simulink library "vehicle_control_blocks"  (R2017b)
settings: Solver=ode1  StartTime=0.0  StopTime=Inf  FixedStep=0.001  RelTol=1e-3  EnableMultiTasking=on
PostLoadFcn:
  | , if any(exist('dsrtsu_mdlpostloadfcn', 'file') == [2, 3, 6]), try dsrtsu_mdlpostloadfcn('Execute', bdroot); catch fprintf('Error in PostLoadFcn (dsrtsu_mdlpostloadfcn) for model "%s":\n %s\n', bdroot, lasterr); end, end,
undefined symbols (not defined in the file or in its folder): ACCEL_KI, ACCEL_KP, ACCEL_MAX, ACCEL_TAU, ACCEL_TS, BRAKE_DEADBAND, DECEL_MAX, FUEL_CAPACITY, GAS_DENSITY, MAX_LATERAL_ACCEL, MAX_STEERING_WHEEL_ANGLE, MIN_SPEED, SPEED_KI, SPEED_KP, SPEED_TS, STEER_KP, STEERING_RATIO, VEHICLE_MASS, WHEEL_RADIUS, WHEELBASE
libraries: simulink x5

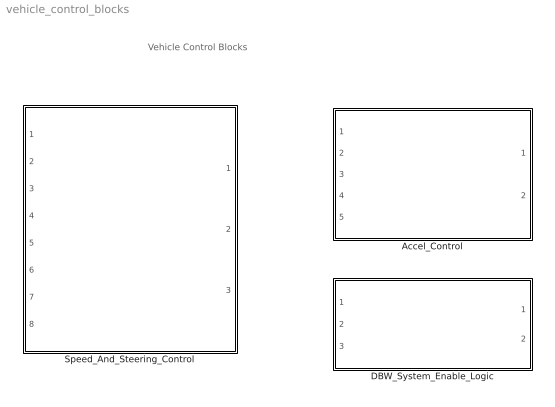
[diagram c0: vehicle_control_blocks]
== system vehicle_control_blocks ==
  note: Vehicle Control Blocks
  Accel_Control : Subsystem  InitFcn=accel_controller_config_init
  DBW_System_Enable_Logic : Subsystem
  Speed_And_Steering_Control : Subsystem  InitFcn=speed_controller_config_init

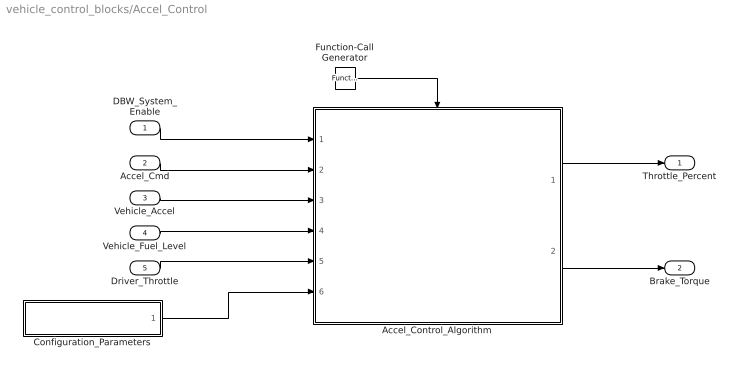
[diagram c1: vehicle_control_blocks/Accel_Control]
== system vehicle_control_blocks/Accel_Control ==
  DBW_System_Enable : Inport
  Accel_Cmd : Inport  Port=2
  Vehicle_Accel : Inport  Port=3
  Vehicle_Fuel_Level : Inport  Port=4
  Driver_Throttle : Inport  Port=5
  Accel_Control_Algorithm : Subsystem
  Configuration_Parameters : Subsystem
  Function-Call Generator : simulink/Ports & Subsystems/Function-Call Generator  sample_time=ACCEL_TS  numberOfIterations=1
  Throttle_Percent : Outport
  Brake_Torque : Outport  Port=2
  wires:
  Configuration_Parameters/1(Calibration_Parameters_Bus) -> Accel_Control_Algorithm/6(Calibration_Parameters_Bus)
  Vehicle_Fuel_Level/1 -> Accel_Control_Algorithm/4(Vehicle_Fuel_Level)
  Accel_Control_Algorithm/1(Throttle_Percent) -> Throttle_Percent/1
  Accel_Control_Algorithm/2(Brake_Torque) -> Brake_Torque/1
  Accel_Cmd/1 -> Accel_Control_Algorithm/2(Accel_Cmd)
  Vehicle_Accel/1 -> Accel_Control_Algorithm/3(Vehicle_Accel)
  Function-Call Generator/1 -> Accel_Control_Algorithm/Trigger
  DBW_System_Enable/1 -> Accel_Control_Algorithm/1(DBW_System_Enable)
  Driver_Throttle/1 -> Accel_Control_Algorithm/5(Driver_Throttle)

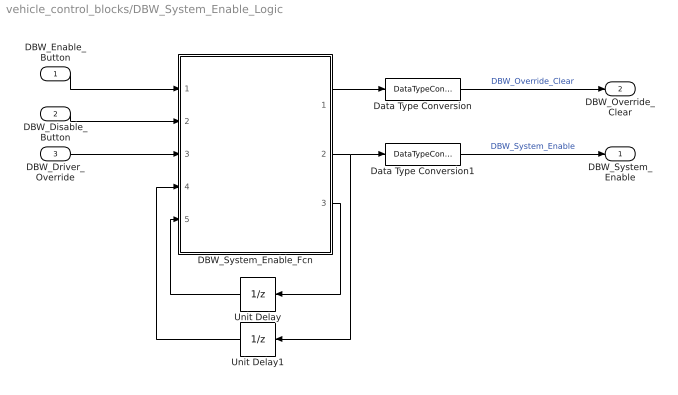
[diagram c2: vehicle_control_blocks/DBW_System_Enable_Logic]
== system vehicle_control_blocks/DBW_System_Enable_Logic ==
  DBW_Enable_Button : Inport
  DBW_Disable_Button : Inport  Port=2
  DBW_Driver_Override : Inport  Port=3
  DBW_System_Enable_Fcn : MATLAB Function  TreatAsAtomicUnit=on
  Data Type Conversion : DataTypeConversion  OutDataTypeStr=boolean
  Data Type Conversion1 : DataTypeConversion  OutDataTypeStr=boolean
  Unit Delay : UnitDelay  SampleTime=-1
  Unit Delay1 : UnitDelay  SampleTime=-1
  DBW_System_Enable : Outport
  DBW_Override_Clear : Outport  Port=2
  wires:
  DBW_Enable_Button/1 -> DBW_System_Enable_Fcn/1(enable_button)
  DBW_Disable_Button/1 -> DBW_System_Enable_Fcn/2(disable_button)
  DBW_Driver_Override/1 -> DBW_System_Enable_Fcn/3(driver_override)
  DBW_System_Enable_Fcn/3(state) -> Unit Delay/1
  DBW_System_Enable_Fcn/2(enable) -> Unit Delay1/1, Data Type Conversion1/1
  Unit Delay/1 -> DBW_System_Enable_Fcn/5(state_prev)
  Unit Delay1/1 -> DBW_System_Enable_Fcn/4(enable_prev)
  DBW_System_Enable_Fcn/1(clear_override) -> Data Type Conversion/1
  Data Type Conversion/1 -> DBW_Override_Clear/1  "DBW_Override_Clear"
  Data Type Conversion1/1 -> DBW_System_Enable/1  "DBW_System_Enable"

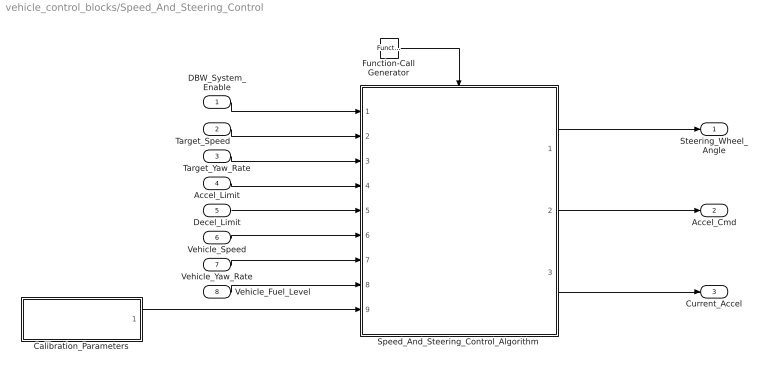
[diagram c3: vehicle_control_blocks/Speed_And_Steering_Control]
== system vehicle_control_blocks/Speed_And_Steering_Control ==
  DBW_System_Enable : Inport
  Target_Speed : Inport  Port=2
  Target_Yaw_Rate : Inport  Port=3
  Accel_Limit : Inport  Port=4
  Decel_Limit : Inport  Port=5
  Vehicle_Speed : Inport  Port=6
  Vehicle_Yaw_Rate : Inport  Port=7
  Vehicle_Fuel_Level : Inport  Port=8
  Calibration_Parameters : Subsystem
  Function-Call Generator : simulink/Ports & Subsystems/Function-Call Generator  sample_time=SPEED_TS  numberOfIterations=1
  Speed_And_Steering_Control_Algorithm : Subsystem
  Steering_Wheel_Angle : Outport
  Accel_Cmd : Outport  Port=2
  Current_Accel : Outport  Port=3
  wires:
  Calibration_Parameters/1(Calibration_Parameters_Bus) -> Speed_And_Steering_Control_Algorithm/9(Calibration_Parameters_Bus)
  Speed_And_Steering_Control_Algorithm/2(Accel_Cmd) -> Accel_Cmd/1
  Target_Speed/1 -> Speed_And_Steering_Control_Algorithm/2(Target_Speed)
  Target_Yaw_Rate/1 -> Speed_And_Steering_Control_Algorithm/3(Target_Yaw_Rate)
  Vehicle_Speed/1 -> Speed_And_Steering_Control_Algorithm/6(Vehicle_Speed)
  Speed_And_Steering_Control_Algorithm/1(Steering_Wheel_Angle) -> Steering_Wheel_Angle/1
  Vehicle_Yaw_Rate/1 -> Speed_And_Steering_Control_Algorithm/7(Vehicle_Yaw_Rate)
  Function-Call Generator/1 -> Speed_And_Steering_Control_Algorithm/Trigger
  Speed_And_Steering_Control_Algorithm/3(Current_Accel) -> Current_Accel/1
  Accel_Limit/1 -> Speed_And_Steering_Control_Algorithm/4(Accel_Limit)
  Decel_Limit/1 -> Speed_And_Steering_Control_Algorithm/5(Decel_Limit)
  DBW_System_Enable/1 -> Speed_And_Steering_Control_Algorithm/1(DBW_System_Enable)
  Vehicle_Fuel_Level/1 -> Speed_And_Steering_Control_Algorithm/8(Vehicle_Fuel_Level)

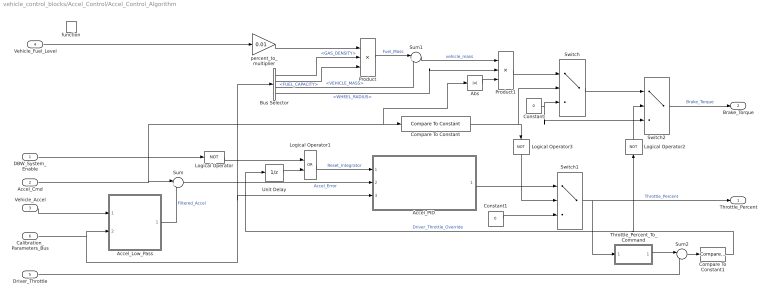
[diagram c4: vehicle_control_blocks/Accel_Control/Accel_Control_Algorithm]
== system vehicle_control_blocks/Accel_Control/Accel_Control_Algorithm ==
  DBW_System_Enable : Inport
  Accel_Cmd : Inport  Port=2
  Vehicle_Accel : Inport  Port=3
  Vehicle_Fuel_Level : Inport  Port=4
  Driver_Throttle : Inport  Port=5
  Calibration_Parameters_Bus : Inport  Port=6
  function : TriggerPort  TriggerType=function-call  VariantControl=Variant
  Abs : Abs
  Accel_Low_Pass : Subsystem  TreatAsAtomicUnit=on
  Accel_PID : Subsystem  TreatAsAtomicUnit=on
  Bus Selector : BusSelector  OutputSignals=GAS_DENSITY,FUEL_CAPACITY,VEHICLE_MASS,WHEEL_RADIUS
  Compare To Constant : simulink/Logic and Bit Operations/Compare To Constant  relop=<  const=-BRAKE_DEADBAND  OutDataTypeStr=uint8
  Compare To Constant1 : simulink/Logic and Bit Operations/Compare To Constant  relop=>=  const=0.1  OutDataTypeStr=uint8
  Constant : Constant  Value=0
  Constant1 : Constant  Value=0
  Logical Operator : Logic  Operator=NOT  AllPortsSameDT=off  OutDataTypeStr=boolean
  Logical Operator1 : Logic  Operator=OR  AllPortsSameDT=off  OutDataTypeStr=boolean
  Logical Operator2 : Logic  Operator=NOT  AllPortsSameDT=off  OutDataTypeStr=boolean
  Logical Operator3 : Logic  Operator=NOT  AllPortsSameDT=off  OutDataTypeStr=boolean
  Product : Product  Inputs=3
  Product1 : Product  Inputs=3
  Sum : Sum  Inputs=|+-
  Sum1 : Sum  Inputs=|++
  Sum2 : Sum  Inputs=|-+
  Switch : Switch  Criteria=u2 ~= 0
  Switch1 : Switch  Criteria=u2 ~= 0
  Switch2 : Switch  Criteria=u2 ~= 0
  Throttle_Percent_To_Command : MATLAB Function  TreatAsAtomicUnit=on
  Unit Delay : UnitDelay  SampleTime=-1
  percent_to_multiplier : Gain  Gain=0.01
  Throttle_Percent : Outport
  Brake_Torque : Outport  Port=2
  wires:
  Calibration_Parameters_Bus/1 -> Accel_Low_Pass/2(Config_Params), Accel_PID/3(Config_Params), Bus Selector/1
  Accel_Cmd/1 -> Sum/1, Compare To Constant/1, Abs/1
  Accel_Low_Pass/1(Y) -> Sum/2  "Filtered_Accel"
  Sum/1 -> Accel_PID/2(Accel_Error)  "Accel_Error"
  Bus Selector/1 -> Product/2  "<GAS_DENSITY>"
  Bus Selector/2 -> Product/3  "<FUEL_CAPACITY>"
  Bus Selector/3 -> Sum1/2  "<VEHICLE_MASS>"
  percent_to_multiplier/1 -> Product/1
  Product/1 -> Sum1/1  "Fuel_Mass"
  Vehicle_Fuel_Level/1 -> percent_to_multiplier/1
  Sum1/1 -> Product1/1  "vehicle_mass"
  Bus Selector/4 -> Product1/2  "<WHEEL_RADIUS>"
  Vehicle_Accel/1 -> Accel_Low_Pass/1(U)
  Accel_PID/1(Throttle_Percent) -> Switch1/1
  Compare To Constant/1 -> Switch/2, Logical Operator3/1
  Product1/1 -> Switch/1
  Constant/1 -> Switch/3, Switch2/3
  DBW_System_Enable/1 -> Logical Operator/1
  Logical Operator1/1 -> Accel_PID/1(Reset_Integrator)  "Reset_Integrator"
  Logical Operator/1 -> Logical Operator1/1
  Abs/1 -> Product1/3
  Driver_Throttle/1 -> Sum2/2
  Sum2/1 -> Compare To Constant1/1
  Throttle_Percent_To_Command/1(cmd) -> Sum2/1
  Compare To Constant1/1 -> Logical Operator2/1, Unit Delay/1  "Driver_Throttle_Override"
  Switch2/1 -> Brake_Torque/1  "Brake_Torque"
  Switch/1 -> Switch2/1
  Logical Operator2/1 -> Switch2/2
  Switch1/1 -> Throttle_Percent/1, Throttle_Percent_To_Command/1(pct)  "Throttle_Percent"
  Constant1/1 -> Switch1/3
  Logical Operator3/1 -> Switch1/2
  Unit Delay/1 -> Logical Operator1/2

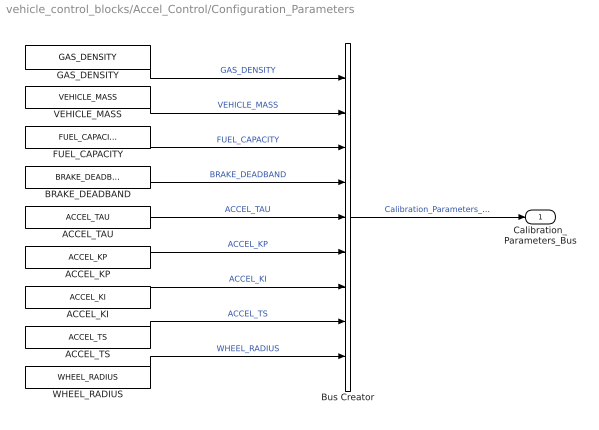
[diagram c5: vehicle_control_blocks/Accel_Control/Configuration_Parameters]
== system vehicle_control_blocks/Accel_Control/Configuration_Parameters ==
  ACCEL_KI : Constant  Value=ACCEL_KI
  ACCEL_KP : Constant  Value=ACCEL_KP
  ACCEL_TAU : Constant  Value=ACCEL_TAU
  ACCEL_TS : Constant  Value=ACCEL_TS
  BRAKE_DEADBAND : Constant  Value=BRAKE_DEADBAND
  Bus Creator : BusCreator  Inputs=9
  FUEL_CAPACITY : Constant  Value=FUEL_CAPACITY
  GAS_DENSITY : Constant  Value=GAS_DENSITY
  VEHICLE_MASS : Constant  Value=VEHICLE_MASS
  WHEEL_RADIUS : Constant  Value=WHEEL_RADIUS
  Calibration_Parameters_Bus : Outport
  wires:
  GAS_DENSITY/1 -> Bus Creator/1  "GAS_DENSITY"
  VEHICLE_MASS/1 -> Bus Creator/2  "VEHICLE_MASS"
  FUEL_CAPACITY/1 -> Bus Creator/3  "FUEL_CAPACITY"
  BRAKE_DEADBAND/1 -> Bus Creator/4  "BRAKE_DEADBAND"
  ACCEL_TAU/1 -> Bus Creator/5  "ACCEL_TAU"
  ACCEL_KP/1 -> Bus Creator/6  "ACCEL_KP"
  ACCEL_KI/1 -> Bus Creator/7  "ACCEL_KI"
  Bus Creator/1 -> Calibration_Parameters_Bus/1  "Calibration_Parameters_Bus"
  ACCEL_TS/1 -> Bus Creator/8  "ACCEL_TS"
  WHEEL_RADIUS/1 -> Bus Creator/9  "WHEEL_RADIUS"

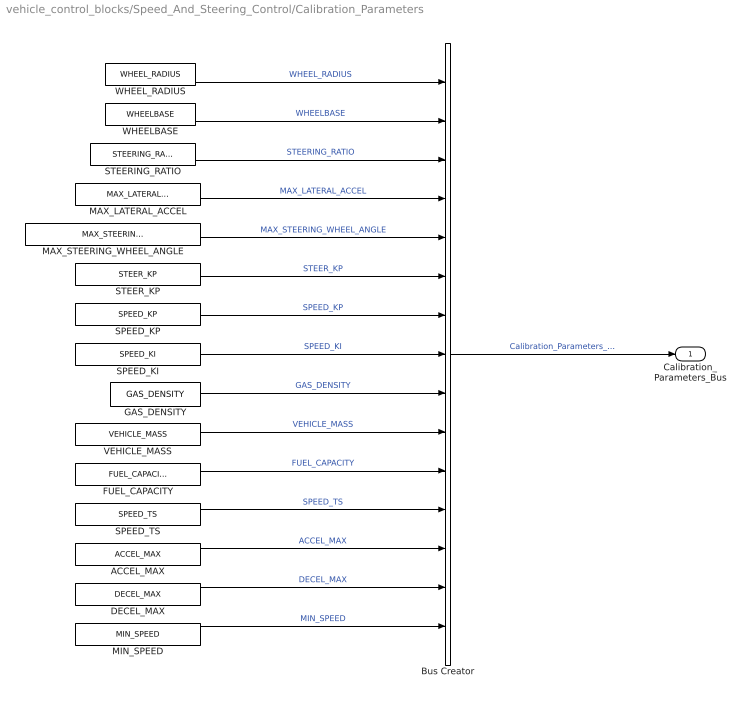
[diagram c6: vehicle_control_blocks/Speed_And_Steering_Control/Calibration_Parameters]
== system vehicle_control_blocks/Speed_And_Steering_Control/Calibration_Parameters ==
  ACCEL_MAX : Constant  Value=ACCEL_MAX
  Bus Creator : BusCreator  Inputs=15
  DECEL_MAX : Constant  Value=DECEL_MAX
  FUEL_CAPACITY : Constant  Value=FUEL_CAPACITY
  GAS_DENSITY : Constant  Value=GAS_DENSITY
  MAX_LATERAL_ACCEL : Constant  Value=MAX_LATERAL_ACCEL
  MAX_STEERING_WHEEL_ANGLE : Constant  Value=MAX_STEERING_WHEEL_ANGLE
  MIN_SPEED : Constant  Value=MIN_SPEED
  SPEED_KI : Constant  Value=SPEED_KI
  SPEED_KP : Constant  Value=SPEED_KP
  SPEED_TS : Constant  Value=SPEED_TS
  STEERING_RATIO : Constant  Value=STEERING_RATIO
  STEER_KP : Constant  Value=STEER_KP
  VEHICLE_MASS : Constant  Value=VEHICLE_MASS
  WHEELBASE : Constant  Value=WHEELBASE
  WHEEL_RADIUS : Constant  Value=WHEEL_RADIUS
  Calibration_Parameters_Bus : Outport
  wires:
  Bus Creator/1 -> Calibration_Parameters_Bus/1  "Calibration_Parameters_Bus"
  WHEEL_RADIUS/1 -> Bus Creator/1  "WHEEL_RADIUS"
  WHEELBASE/1 -> Bus Creator/2  "WHEELBASE"
  STEERING_RATIO/1 -> Bus Creator/3  "STEERING_RATIO"
  MAX_LATERAL_ACCEL/1 -> Bus Creator/4  "MAX_LATERAL_ACCEL"
  MAX_STEERING_WHEEL_ANGLE/1 -> Bus Creator/5  "MAX_STEERING_WHEEL_ANGLE"
  STEER_KP/1 -> Bus Creator/6  "STEER_KP"
  SPEED_KP/1 -> Bus Creator/7  "SPEED_KP"
  SPEED_KI/1 -> Bus Creator/8  "SPEED_KI"
  GAS_DENSITY/1 -> Bus Creator/9  "GAS_DENSITY"
  VEHICLE_MASS/1 -> Bus Creator/10  "VEHICLE_MASS"
  FUEL_CAPACITY/1 -> Bus Creator/11  "FUEL_CAPACITY"
  SPEED_TS/1 -> Bus Creator/12  "SPEED_TS"
  ACCEL_MAX/1 -> Bus Creator/13  "ACCEL_MAX"
  DECEL_MAX/1 -> Bus Creator/14  "DECEL_MAX"
  MIN_SPEED/1 -> Bus Creator/15  "MIN_SPEED"

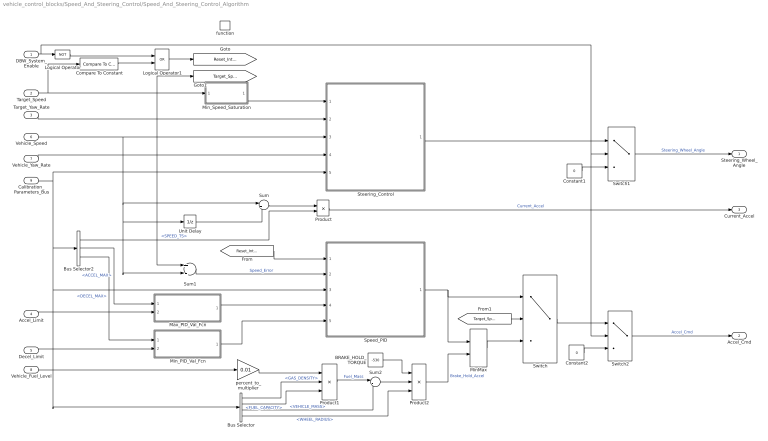
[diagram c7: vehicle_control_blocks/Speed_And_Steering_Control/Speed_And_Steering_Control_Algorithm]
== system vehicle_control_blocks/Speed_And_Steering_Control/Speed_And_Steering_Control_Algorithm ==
  DBW_System_Enable : Inport
  Target_Speed : Inport  Port=2
  Target_Yaw_Rate : Inport  Port=3
  Accel_Limit : Inport  Port=4
  Decel_Limit : Inport  Port=5
  Vehicle_Speed : Inport  Port=6
  Vehicle_Yaw_Rate : Inport  Port=7
  Vehicle_Fuel_Level : Inport  Port=8
  Calibration_Parameters_Bus : Inport  Port=9
  function : TriggerPort  TriggerType=function-call  VariantControl=Variant
  BRAKE_HOLD_TORQUE : Constant  Value=-530
  Bus Selector : BusSelector  OutputSignals=GAS_DENSITY,FUEL_CAPACITY,VEHICLE_MASS,WHEEL_RADIUS
  Bus Selector2 : BusSelector  OutputSignals=SPEED_TS,ACCEL_MAX,DECEL_MAX
  Compare To Constant : simulink/Logic and Bit Operations/Compare To Constant  relop=<=  const=0.447  OutDataTypeStr=uint8
  Constant1 : Constant  Value=0
  Constant2 : Constant  Value=0
  Logical Operator : Logic  Operator=NOT  AllPortsSameDT=off  OutDataTypeStr=boolean
  Logical Operator1 : Logic  Operator=OR  AllPortsSameDT=off  OutDataTypeStr=boolean
  Max_PID_Val_Fcn : MATLAB Function  TreatAsAtomicUnit=on
  MinMax : MinMax  Inputs=2
  Min_PID_Val_Fcn : MATLAB Function  TreatAsAtomicUnit=on
  Min_Speed_Saturation : MATLAB Function  TreatAsAtomicUnit=on
  Product : Product  Inputs=*/
  Product1 : Product  Inputs=3
  Product2 : Product  Inputs=*//
  Speed_PID : Subsystem  TreatAsAtomicUnit=on
  Steering_Control : Subsystem
  Sum : Sum  Inputs=|+-
  Sum1 : Sum  Inputs=+-
  Sum2 : Sum  Inputs=|++
  Switch : Switch  Criteria=u2 > Threshold  Threshold=0.01
  Switch1 : Switch  Criteria=u2 ~= 0  Threshold=0.01
  Switch2 : Switch  Criteria=u2 ~= 0  Threshold=0.01
  Unit Delay : UnitDelay  SampleTime=-1
  percent_to_multiplier : Gain  Gain=0.01
  Steering_Wheel_Angle : Outport
  Accel_Cmd : Outport  Port=2
  Current_Accel : Outport  Port=3
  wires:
  Target_Yaw_Rate/1 -> Steering_Control/2(Target_Yaw_Rate)
  Calibration_Parameters_Bus/1 -> Steering_Control/5(Calibration_Parameters_Bus), Bus Selector2/1, Speed_PID/3(Calibration_Parameters_Bus), Bus Selector/1
  Vehicle_Speed/1 -> Steering_Control/3(Vehicle_Speed), Sum/1, Unit Delay/1, Sum1/2
  Target_Speed/1 -> Compare To Constant/1, Sum1/1, [Target_Speed], Min_Speed_Saturation/1(u)
  Vehicle_Yaw_Rate/1 -> Steering_Control/4(Vehicle_Yaw_Rate)
  Bus Selector2/2 -> Max_PID_Val_Fcn/1(accel_max)  "<ACCEL_MAX>"
  Bus Selector2/3 -> Min_PID_Val_Fcn/1(decel_max)  "<DECEL_MAX>"
  Decel_Limit/1 -> Min_PID_Val_Fcn/2(decel_limit)
  Accel_Limit/1 -> Max_PID_Val_Fcn/2(accel_limit)
  Min_PID_Val_Fcn/1(min_pid_val) -> Speed_PID/5(min_pid_val)
  Max_PID_Val_Fcn/1(max_pid_val) -> Speed_PID/4(max_pid_val)
  Unit Delay/1 -> Sum/2
  Sum/1 -> Product/1
  Bus Selector2/1 -> Product/2  "<SPEED_TS>"
  Product/1 -> Current_Accel/1  "Current_Accel"
  Sum1/1 -> Speed_PID/2(Speed_Error)  "Speed_Error"
  DBW_System_Enable/1 -> Logical Operator/1, Switch2/2, Switch1/2
  Logical Operator/1 -> Logical Operator1/1
  Logical Operator1/1 -> [Reset_Integrator]
  [Reset_Integrator] -> Speed_PID/1(Reset_Integrator)
  [Target_Speed] -> Switch/2
  Speed_PID/1(Accel_Cmd) -> Switch/1, MinMax/1
  MinMax/1 -> Switch/3
  Bus Selector/1 -> Product1/2  "<GAS_DENSITY>"
  Bus Selector/2 -> Product1/3  "<FUEL_CAPACITY>"
  Bus Selector/3 -> Sum2/2  "<VEHICLE_MASS>"
  percent_to_multiplier/1 -> Product1/1
  Product1/1 -> Sum2/1  "Fuel_Mass"
  Bus Selector/4 -> Product2/3  "<WHEEL_RADIUS>"
  Vehicle_Fuel_Level/1 -> percent_to_multiplier/1
  BRAKE_HOLD_TORQUE/1 -> Product2/1
  Sum2/1 -> Product2/2
  Product2/1 -> MinMax/2  "Brake_Hold_Accel"
  Min_Speed_Saturation/1(y) -> Steering_Control/1(Target_Speed)
  Steering_Control/1(Steering_Wheel_Angle) -> Switch1/1
  Constant1/1 -> Switch1/3
  Switch1/1 -> Steering_Wheel_Angle/1  "Steering_Wheel_Angle"
  Constant2/1 -> Switch2/3
  Switch/1 -> Switch2/1
  Switch2/1 -> Accel_Cmd/1  "Accel_Cmd"
  Compare To Constant/1 -> Logical Operator1/2

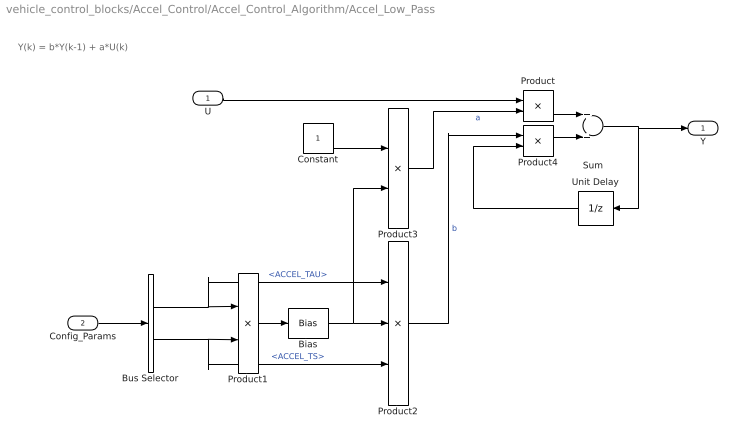
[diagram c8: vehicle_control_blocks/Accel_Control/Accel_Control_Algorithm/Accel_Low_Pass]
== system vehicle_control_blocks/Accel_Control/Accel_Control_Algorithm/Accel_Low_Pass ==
  note: Y(k) = b*Y(k-1) + a*U(k)
  U : Inport
  Config_Params : Inport  Port=2
  Bias : Bias  Bias=1
  Bus Selector : BusSelector  OutputSignals=ACCEL_TAU,ACCEL_TS
  Constant : Constant
  Product : Product
  Product1 : Product  Inputs=*/
  Product2 : Product  Inputs=*//
  Product3 : Product  Inputs=*/
  Product4 : Product
  Sum : Sum
  Unit Delay : UnitDelay  SampleTime=-1
  Y : Outport
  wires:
  Config_Params/1 -> Bus Selector/1
  Sum/1 -> Y/1, Unit Delay/1
  U/1 -> Product/1
  Bus Selector/1 -> Product1/1, Product2/1  "<ACCEL_TAU>"
  Bus Selector/2 -> Product1/2, Product2/3  "<ACCEL_TS>"
  Product1/1 -> Bias/1
  Bias/1 -> Product2/2, Product3/2
  Constant/1 -> Product3/1
  Product3/1 -> Product/2  "a"
  Product2/1 -> Product4/1  "b"
  Product/1 -> Sum/1
  Product4/1 -> Sum/2
  Unit Delay/1 -> Product4/2

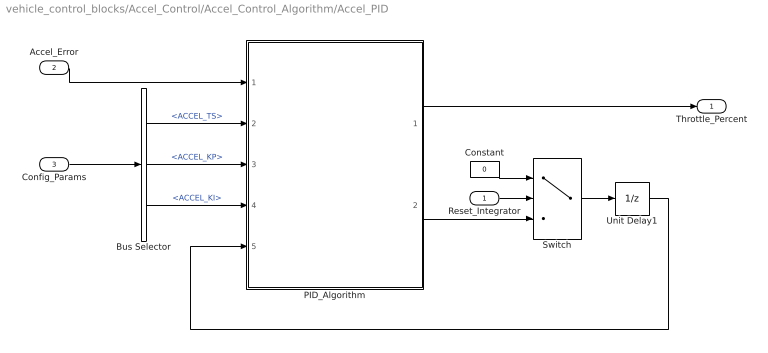
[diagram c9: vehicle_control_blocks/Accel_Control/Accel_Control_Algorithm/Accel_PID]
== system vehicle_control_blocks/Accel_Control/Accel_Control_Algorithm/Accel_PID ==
  Reset_Integrator : Inport
  Accel_Error : Inport  Port=2
  Config_Params : Inport  Port=3
  Bus Selector : BusSelector  OutputSignals=ACCEL_TS,ACCEL_KP,ACCEL_KI
  Constant : Constant  Value=0
  PID_Algorithm : MATLAB Function  TreatAsAtomicUnit=on
  Switch : Switch  Criteria=u2 ~= 0
  Unit Delay1 : UnitDelay  SampleTime=-1
  Throttle_Percent : Outport
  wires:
  Config_Params/1 -> Bus Selector/1
  Accel_Error/1 -> PID_Algorithm/1(error)
  Bus Selector/1 -> PID_Algorithm/2(sample_time)  "<ACCEL_TS>"
  Bus Selector/3 -> PID_Algorithm/4(ki)  "<ACCEL_KI>"
  Bus Selector/2 -> PID_Algorithm/3(kp)  "<ACCEL_KP>"
  PID_Algorithm/1(throttle_percent) -> Throttle_Percent/1
  PID_Algorithm/2(int_val) -> Switch/3
  Switch/1 -> Unit Delay1/1
  Reset_Integrator/1 -> Switch/2
  Constant/1 -> Switch/1
  Unit Delay1/1 -> PID_Algorithm/5(last_int_val)

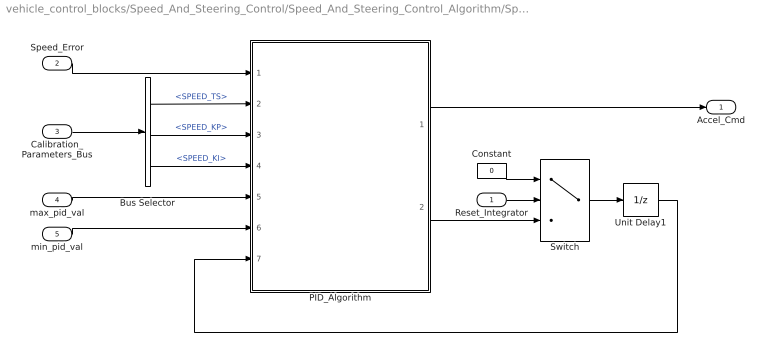
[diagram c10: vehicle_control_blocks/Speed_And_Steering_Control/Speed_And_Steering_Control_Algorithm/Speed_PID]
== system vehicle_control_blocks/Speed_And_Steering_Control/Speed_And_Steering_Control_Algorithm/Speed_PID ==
  Reset_Integrator : Inport
  Speed_Error : Inport  Port=2
  Calibration_Parameters_Bus : Inport  Port=3
  max_pid_val : Inport  Port=4
  min_pid_val : Inport  Port=5
  Bus Selector : BusSelector  OutputSignals=SPEED_TS,SPEED_KP,SPEED_KI
  Constant : Constant  Value=0
  PID_Algorithm : MATLAB Function  TreatAsAtomicUnit=on
  Switch : Switch  Criteria=u2 ~= 0
  Unit Delay1 : UnitDelay  SampleTime=-1
  Accel_Cmd : Outport
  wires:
  Calibration_Parameters_Bus/1 -> Bus Selector/1
  Speed_Error/1 -> PID_Algorithm/1(error)
  Bus Selector/1 -> PID_Algorithm/2(sample_time)  "<SPEED_TS>"
  Bus Selector/3 -> PID_Algorithm/4(ki)  "<SPEED_KI>"
  Bus Selector/2 -> PID_Algorithm/3(kp)  "<SPEED_KP>"
  PID_Algorithm/1(Accel_Cmd) -> Accel_Cmd/1
  PID_Algorithm/2(integrator_val) -> Switch/3
  Switch/1 -> Unit Delay1/1
  Reset_Integrator/1 -> Switch/2
  Constant/1 -> Switch/1
  Unit Delay1/1 -> PID_Algorithm/7(last_integrator_val)
  min_pid_val/1 -> PID_Algorithm/6(min_pid_val)
  max_pid_val/1 -> PID_Algorithm/5(max_pid_val)

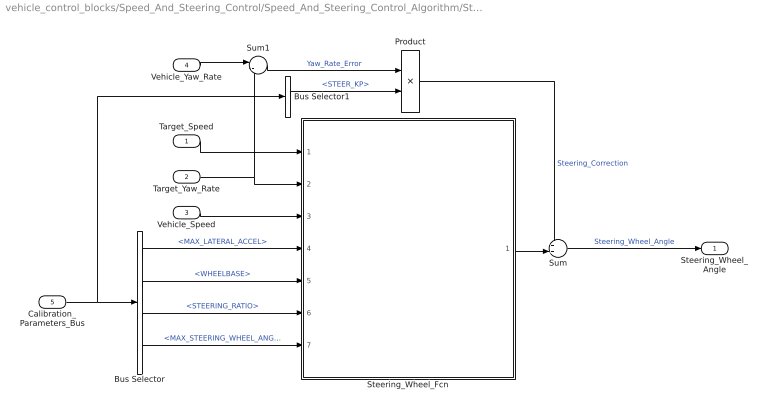
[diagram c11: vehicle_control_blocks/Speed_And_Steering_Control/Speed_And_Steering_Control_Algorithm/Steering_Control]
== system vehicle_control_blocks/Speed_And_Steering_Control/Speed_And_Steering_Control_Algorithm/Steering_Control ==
  Target_Speed : Inport
  Target_Yaw_Rate : Inport  Port=2
  Vehicle_Speed : Inport  Port=3
  Vehicle_Yaw_Rate : Inport  Port=4
  Calibration_Parameters_Bus : Inport  Port=5
  Bus Selector : BusSelector  OutputSignals=MAX_LATERAL_ACCEL,WHEELBASE,STEERING_RATIO,MAX_STEERING_WHEEL_ANGLE
  Bus Selector1 : BusSelector  OutputSignals=STEER_KP
  Product : Product
  Steering_Wheel_Fcn : MATLAB Function  TreatAsAtomicUnit=on
  Sum : Sum  Inputs=++|
  Sum1 : Sum  Inputs=|-+
  Steering_Wheel_Angle : Outport
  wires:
  Target_Speed/1 -> Steering_Wheel_Fcn/1(target_speed)
  Target_Yaw_Rate/1 -> Steering_Wheel_Fcn/2(target_yaw_rate), Sum1/2
  Vehicle_Speed/1 -> Steering_Wheel_Fcn/3(vehicle_speed)
  Calibration_Parameters_Bus/1 -> Bus Selector/1, Bus Selector1/1
  Bus Selector/1 -> Steering_Wheel_Fcn/4(MAX_LATERAL_ACCEL)  "<MAX_LATERAL_ACCEL>"
  Bus Selector/2 -> Steering_Wheel_Fcn/5(WHEELBASE)  "<WHEELBASE>"
  Bus Selector/3 -> Steering_Wheel_Fcn/6(STEERING_RATIO)  "<STEERING_RATIO>"
  Bus Selector/4 -> Steering_Wheel_Fcn/7(MAX_STEERING_WHEEL_ANGLE)  "<MAX_STEERING_WHEEL_ANGLE>"
  Vehicle_Yaw_Rate/1 -> Sum1/1
  Bus Selector1/1 -> Product/2  "<STEER_KP>"
  Sum1/1 -> Product/1  "Yaw_Rate_Error"
  Steering_Wheel_Fcn/1(wheel_angle) -> Sum/2
  Product/1 -> Sum/1  "Steering_Correction"
  Sum/1 -> Steering_Wheel_Angle/1  "Steering_Wheel_Angle"

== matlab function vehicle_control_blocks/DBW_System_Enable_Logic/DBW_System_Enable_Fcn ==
%% Function Name: DBW_System_Enable_Fcn
% 
% Description: Generates a driver override clear signal and an enable
%   signal in response to steering wheel button presses.
%
% Assumptions: None
%
% Inputs:                                           Size
%   Boolean signal to enable DBW control            1x1
%   Boolean signal to disable DBW control           1x1
%   Boolean driver override status                  1x1
%   Previous enable signal output                   1x1
%   Previous state                                  1x1
%
% Outputs:                                          Size
%   Clear signal to be sent to each DBW interface   1x1
%   Enable signal indicating DBW control is ready   1x1
%   Internal state of the system enable logic       1x1
%
% $Revision: 1.0$
% $Author: Micho Radovnikovich$
% $Date: August 3, 2015$
%
%-----------------------------------------

function [clear_override, enable, state]  = dbw_enable(enable_button, disable_button,...
    driver_override, enable_prev, state_prev)

state = state_prev;
clear_override = 0;

% Detect if the driver is depressing proper buttons to signal request for
% enabling or disabling the DBW system.
if enable_button == 1
    state = 1;
elseif disable_button == 1
    state = 0;
end

if state == 1
    if driver_override == 0
        % If DBW was already enabled or a new request to do so has appeared, 
        % and there are no driver overrides, enable DBW.
        enable = 1;
    else
        % DRIVER OVERRIDE EXISTS.
        
        % The following IF condition exists because when the user initially presses the 
        % buttons, there will likely already be an override condition set, 
        % and without this IF block, the logic will instantly reset 'state' 
        % to zero.
        if enable_prev == 1  
            state = 0;
        end
        enable = 0;
        
        % The following line is to clear an existing driver override 
        % condition when the user presses the enable button(s).  After setting 
        % "clear_override" to 1, the next cycle through this state machine should see 
        % that "driver_override" is 0.  However, the driver override condition persists 
        % while the user holds the brake pedal down.  Therefore, if the driver 
        % holds the brakes, then hits the enable button, the state machine will 
        % keep hitting the 'en = 0; clear = 1;' lines until the user releases 
        % the brakes and the driver override is cleared.  At this point, the 
        % state machine hits the 'en = 1' line and the DBW system is enabled.
        clear_override = 1;
    end
else
    % State was previously disabled, and no new request by the driver has
    % been received to enable it; or the driver has requested to disable.
    enable = 0;
end

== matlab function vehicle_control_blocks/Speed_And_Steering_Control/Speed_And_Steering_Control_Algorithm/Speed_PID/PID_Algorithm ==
function [Accel_Cmd, integrator_val] = fcn(error, sample_time, kp, ki, ...
    max_pid_val, min_pid_val, last_integrator_val)

integrator_val = last_integrator_val;
new_integrator_val = last_integrator_val + error * sample_time;

Accel_Cmd = kp * error + ki * last_integrator_val;
if Accel_Cmd > max_pid_val
    Accel_Cmd = max_pid_val;
elseif Accel_Cmd < min_pid_val
    Accel_Cmd = min_pid_val;
else
    integrator_val = new_integrator_val;
end

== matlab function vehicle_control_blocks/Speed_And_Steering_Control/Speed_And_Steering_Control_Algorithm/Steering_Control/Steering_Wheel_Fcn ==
function wheel_angle = fcn(target_speed, target_yaw_rate, vehicle_speed, ...
    MAX_LATERAL_ACCEL, WHEELBASE, STEERING_RATIO, MAX_STEERING_WHEEL_ANGLE)

%% Limit yaw rate control if speed control error is large 
if abs(target_speed) > 0
    omega_z = target_yaw_rate * vehicle_speed / target_speed;
else    
    omega_z = 0;   
end

%% Saturate yaw rate control to limit lateral acceleration
if abs(vehicle_speed) > 0.1
   max_yaw_rate = abs(MAX_LATERAL_ACCEL / vehicle_speed);
   if omega_z > max_yaw_rate
       omega_z = max_yaw_rate;
   elseif omega_z < -max_yaw_rate
       omega_z = -max_yaw_rate;
   end
end

%% Compute steering wheel angle to implement yaw rate command
% Use minimum of 4 mph to compute turning radius
turning_radius = max(vehicle_speed, 1.78816) / omega_z; 
if ~isfinite(turning_radius)
    wheel_angle = 0;
else
    wheel_angle = atan(WHEELBASE / turning_radius) * STEERING_RATIO;
end

%% Saturate steering wheel angle within physical limits
if wheel_angle > MAX_STEERING_WHEEL_ANGLE
    wheel_angle = MAX_STEERING_WHEEL_ANGLE;
elseif wheel_angle < -MAX_STEERING_WHEEL_ANGLE
    wheel_angle = -MAX_STEERING_WHEEL_ANGLE;
end

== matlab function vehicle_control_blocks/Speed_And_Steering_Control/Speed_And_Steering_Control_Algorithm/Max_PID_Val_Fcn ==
function max_pid_val = fcn(accel_max, accel_limit)

if accel_max == 0 && accel_limit == 0
    max_pid_val = 9.8;
elseif accel_max == 0
    max_pid_val = min(accel_limit, 9.8);
elseif accel_limit == 0
    max_pid_val = min(accel_max, 9.8);
else
    max_pid_val = min(accel_max, min(accel_limit, 9.8));
end

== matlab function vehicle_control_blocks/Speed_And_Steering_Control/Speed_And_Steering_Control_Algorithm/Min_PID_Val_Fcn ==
function min_pid_val = fcn(decel_max, decel_limit)

if decel_max == 0 && decel_limit == 0
    min_pid_val = -9.8;
elseif decel_max == 0
    min_pid_val = -min(decel_limit, 9.8);
elseif decel_limit == 0
    min_pid_val = -min(decel_max, 9.8);
else
    min_pid_val = -min(decel_max, min(decel_limit, 9.8));
end

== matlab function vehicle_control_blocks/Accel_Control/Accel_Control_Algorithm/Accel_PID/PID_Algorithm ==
function [throttle_percent, int_val] = fcn(error, sample_time, kp, ki, last_int_val)

int_val = last_int_val;
new_int_val = last_int_val + error * sample_time;

throttle_percent = kp * error + ki * last_int_val;
if throttle_percent > 1.0
    throttle_percent = 1.0;
elseif throttle_percent < 0
    throttle_percent = 0;
else
    int_val = new_int_val;
end

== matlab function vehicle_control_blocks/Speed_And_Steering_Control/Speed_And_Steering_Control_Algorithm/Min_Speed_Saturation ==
function y = fcn(u)

if (u > 0.01) && (u < 2.23)
    y = 2.23;
else
    y = u;
end

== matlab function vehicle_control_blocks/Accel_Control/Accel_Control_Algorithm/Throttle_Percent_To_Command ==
function cmd = fcn(pct)

cmd = 0.15 + pct * (0.8 - 0.15);
